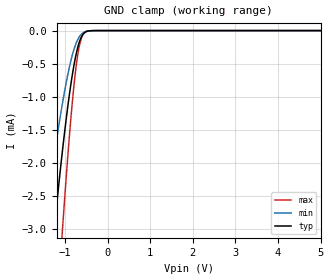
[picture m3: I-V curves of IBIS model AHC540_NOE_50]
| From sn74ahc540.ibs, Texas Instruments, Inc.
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[Model]   AHC540_NOE_50
Model_type  Input
Vinl = 1.65
Vinh = 3.85
| variable   typ   min   max
C_comp   0.66pF   0.58pF   0.75pF
[Temperature Range]   40   100   -40
| Ambient temperature   25   85   -40
[Voltage range]   5   4.5   5.5
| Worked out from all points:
|   GND clamp passes 1 mA (typ) near -0.91 V on its own axis
[GND Clamp]
| AHC540_NOE_50
|   Voltage   I(typ)   I(min)   I(max)
-5V       -39.52mA   -26.01mA   -50.56mA
-1.5V     -4.736mA   -3.022mA   -7.496mA
-1.27V    -3.11mA    -1.953mA   -5.058mA
-1.245V   -2.945mA   -1.845mA   -4.803mA
-1.07V    -1.866mA   -1.133mA   -3.091mA
-1.05V    -1.752mA   -1.058mA   -2.906mA
-875mV    -862.4uA   -486.5uA   -1.416mA
-765mV    -435.2uA   -233.4uA   -674.8uA
-665mV    -173.7uA   -94.05uA   -235.2uA
-615mV    -93.83uA   -53.67uA   -114.8uA
-545mV    -32.81uA   -20.86uA   -33.5uA
5V        15.07nA    1.006nA    138.2nA
